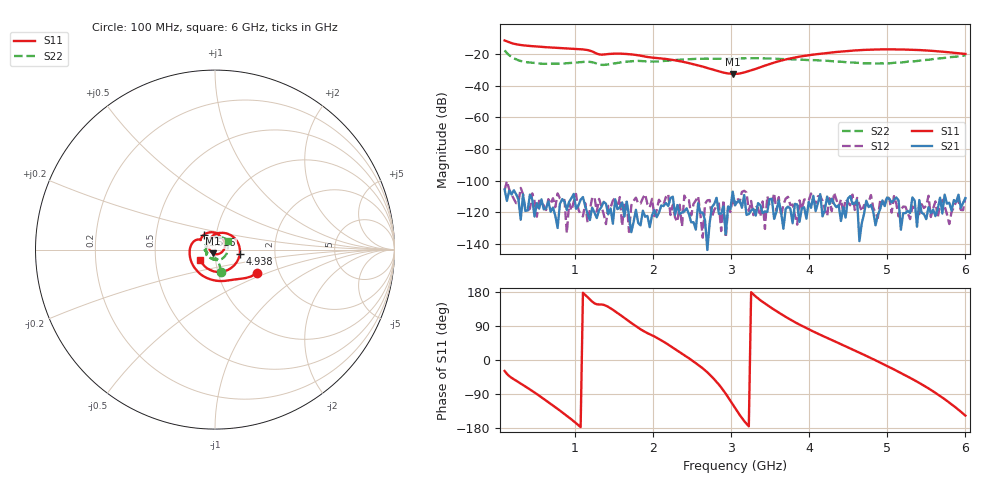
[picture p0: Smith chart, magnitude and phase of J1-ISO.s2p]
!Agilent Technologies,E8364B,MY43040379,A.07.50.67
!Agilent E8364B: A.07.50.67
!Date: Tuesday, March 24, 2026 11:03:56
!Correction: S11(Full 2 Port(1,2))
!S21(Full 2 Port(1,2))
!S12(Full 2 Port(1,2))
!S22(Full 2 Port(1,2))
!S2P File: Measurements: S11, S21, S12, S22:
# Hz S  dB  R 50
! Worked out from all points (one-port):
!   201 points, 100 MHz to 6 GHz, reference 50 ohm
!   lowest |S11| = -32.6 dB at 3.021 GHz (marker M1), VSWR 1.05, Z = 48.9 - j2.06 ohm
!   |S11| at or under -10 dB: start of sweep to end of sweep
!   S11 on the Smith chart (normalised r, x): 100 MHz: 1.54, -0.43; 1.516 GHz: 0.87, +0.14; 4.938 GHz: 1.32, -0.06; 6 GHz: 0.84, -0.09
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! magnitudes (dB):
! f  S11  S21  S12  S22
! 100 MHz  -11.4  -105.6  -106.1  -17.7
! 218 MHz  -13.5  -106.1  -111.6  -22.7
! 365.5 MHz  -14.7  -119.2  -117.9  -25.1
! 601.5 MHz  -15.6  -118.2  -115.6  -26.2
! 1.103 GHz  -17.1  -110.4  -122.6  -25.0
! 1.221 GHz  -18.4  -117.0  -110.9  -25.2
! 1.31 GHz  -20.2  -118.7  -111.6  -26.6
! 1.516 GHz  -19.8  -111.8  -111.0  -25.9
! 1.782 GHz  -20.6  -118.4  -110.8  -24.4
! 2.076 GHz  -22.7  -120.3  -112.1  -24.7
! 2.401 GHz  -25.1  -119.4  -109.5  -23.5
! 2.902 GHz  -31.8  -116.4  -112.2  -23.0
! 3.021 GHz  -32.6  -106.9  -111.2  -22.9
! 3.05 GHz  -32.5  -115.5  -115.6  -22.9
! 3.227 GHz  -30.8  -121.2  -119.3  -22.6
! 3.64 GHz  -24.2  -120.0  -122.4  -23.2
! 4.053 GHz  -20.4  -109.7  -113.3  -23.8
! 4.525 GHz  -18.0  -109.8  -115.6  -25.4
! 4.938 GHz  -17.1  -112.5  -114.7  -25.9
! 5.027 GHz  -17.1  -111.6  -111.6  -25.9
! 5.498 GHz  -17.7  -124.4  -115.9  -23.8
! 6 GHz  -20.0  -111.1  -110.7  -21.0
